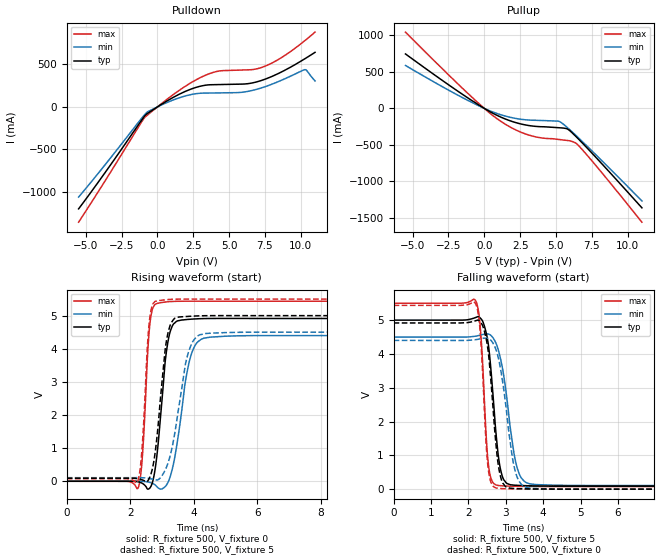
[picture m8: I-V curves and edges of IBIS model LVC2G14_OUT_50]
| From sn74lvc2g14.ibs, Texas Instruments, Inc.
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[Model]   LVC2G14_OUT_50
Model_type  Output
Vref =   0
Rref =   500
Cref =   50p
Vmeas =   2.5
| variable   typ   min   max
C_comp   8.88pF   5.46pF   12.35pF
| C_pullup   9.78pF   5.46pF   12.35pF
| C_pulldown   7.99pF   5.90pF   10.99pF
[Temperature Range]   40   100   -40
| Ambient temperature   25   85   -40
[Voltage range]   5   4.5   5.5
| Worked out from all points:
|   slope of the pulldown table from 0 to 0.75 V, typ, clamps not added: 9.58 ohm
|   slope of the pullup table from 0 to 0.75 V, typ, clamps not added: 9.16 ohm
|   rising waveform, R_fixture 500, V_fixture 0: 20-80 % time 279ps typ, 407ps min, 175ps max; typ from 0 V to 4.91 V
|   falling waveform, R_fixture 500, V_fixture 5: 20-80 % time 230ps typ, 327ps min, 157ps max; typ from 5 V to 0.09 V
|   rising waveform, R_fixture 500, V_fixture 5: 20-80 % time 295ps typ, 449ps min, 179ps max; typ from 0.09 V to 5 V
|   falling waveform, R_fixture 500, V_fixture 0: 20-80 % time 225ps typ, 320ps min, 156ps max; typ from 4.92 V to 0 V
[Pulldown]
| LVC2G14_OUT_50
|   Voltage   I(typ)   I(min)   I(max)
-5.5V     -1.198A    -1.059A    -1.354A
-970mV    -125.1mA   -106.1mA   -141.7mA
-675mV    -74.35mA   -56.48mA   -92.74mA
205mV     22.29mA    16.59mA    27.99mA
1.905V    179.2mA    127mA      238mA
3.285V    253.2mA    162.4mA    367.3mA
4.325V    262.7mA    164.8mA    422.2mA
5.815V    267.8mA    170.7mA    433mA
7.31V     313.8mA    226.4mA    466mA
8.65V     410.1mA    312.7mA    578.8mA
10.28V    565mA      437.4mA    777.7mA
11V       641.2mA    305.2mA    879.1mA
[Pullup]
| LVC2G14_OUT_50
|   Voltage   I(typ)   I(min)   I(max)
-5.5V     745.2mA    587.5mA    1.044A
-1.18V    147.6mA    112.6mA    211.7mA
170mV     -19.98mA   -14.91mA   -29.14mA
1.04V     -109.2mA   -79.97mA   -161.6mA
2.045V    -185.4mA   -131.8mA   -280mA
3.05V     -232.7mA   -158.7mA   -361.3mA
3.945V    -250.5mA   -165.3mA   -402.5mA
5.3V      -265.9mA   -185.4mA   -427.7mA
5.83V     -285.1mA   -268.2mA   -440mA
6.525V    -410.2mA   -394.3mA   -498.1mA
8.085V    -732.8mA   -692.6mA   -852.4mA
11V       -1.361A    -1.267A    -1.557A
[Ramp]
| LVC2G14_OUT_50
| variable   typ   min   max
dV/dt_r   3.09/3.03E-10   2.78/4.45E-10   3.39/1.85E-10
dV/dt_f   3.01/2.40E-10   2.69/3.46E-10   3.33/1.66E-10
R_load = 500
[Rising Waveform]
| LVC2G14_OUT_50
R_fixture =   500
C_fixture =   0
L_fixture =   0
V_fixture =   0
V_fixture_min = 0
V_fixture_max = 0
|   Time   V(typ)   V(min)   V(max)
0s        181.8pV    4.248nV    2.638nV
2.245ns   -16.48mV   1.888mV    -203mV
2.385ns   -66.55mV   -3.025mV   805.7mV
2.615ns   -205.8mV   -34.79mV   4.728V
2.865ns   1.017V     -191.2mV   5.375V
3.095ns   3.58V      -166.1mV   5.41V
3.27ns    4.558V     180.6mV    5.426V
3.855ns   4.889V     3.605V     5.436V
4.315ns   4.912V     4.319V     5.436V
24.99ns   4.914V     4.397V     5.435V
[Falling Waveform]
| LVC2G14_OUT_50
R_fixture =   500
C_fixture =   0
L_fixture =   0
V_fixture =   5
V_fixture_min = 4.5
V_fixture_max = 5.5
|   Time   V(typ)   V(min)   V(max)
0s        5V         4.5V       5.5V
2.2ns     5.081V     4.527V     5.562V
2.325ns   5.055V     4.56V      4.694V
2.475ns   4.629V     4.592V     1.587V
2.54ns    4.228V     4.588V     691.5mV
2.8ns     992.1mV    4.119V     108.8mV
2.945ns   280.6mV    3.36V      95.79mV
3.275ns   115.4mV    758.1mV    84.43mV
3.665ns   98.68mV    152.5mV    79.9mV
24.99ns   89.64mV    107.6mV    78.98mV
[Rising Waveform]
| LVC2G14_OUT_50
R_fixture =   500
C_fixture =   0
L_fixture =   0
V_fixture =   5
V_fixture_min = 4.5
V_fixture_max = 5.5
|   Time   V(typ)   V(min)   V(max)
0s        89.62mV    107.6mV    78.96mV
2.22ns    80.33mV    109.1mV    -36.85mV
2.37ns    44.61mV    106.4mV    982.5mV
2.605ns   102.9mV    83.02mV    4.866V
2.855ns   1.475V     39.11mV    5.449V
3.1ns     3.991V     339.8mV    5.479V
3.265ns   4.732V     809.3mV    5.491V
3.805ns   4.977V     3.809V     5.501V
4.32ns    4.998V     4.453V     5.501V
24.99ns   5V         4.5V       5.5V
[Falling Waveform]
| LVC2G14_OUT_50
R_fixture =   500
C_fixture =   0
L_fixture =   0
V_fixture =   0
V_fixture_min = 0
V_fixture_max = 0
|   Time   V(typ)   V(min)   V(max)
0s        4.917V     4.401V     5.437V
2.19ns    4.981V     4.422V     5.49V
2.315ns   4.952V     4.447V     4.66V
2.465ns   4.502V     4.468V     1.519V
2.525ns   4.12V      4.461V     658.3mV
2.745ns   1.244V     4.109V     33.83mV
2.905ns   213.8mV    3.259V     15.23mV
3.23ns    19.26mV    640.3mV    5.509mV
3.6ns     8.145mV    38.01mV    1.111mV
24.99ns   17.35uV    21.63uV    17.19uV
